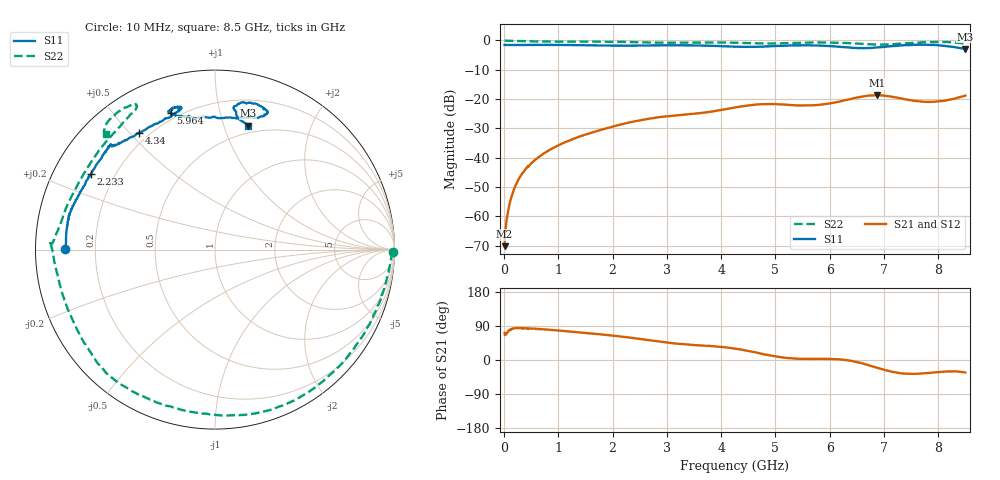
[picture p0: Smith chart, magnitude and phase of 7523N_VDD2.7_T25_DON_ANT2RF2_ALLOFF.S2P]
!Agilent Technologies,E5071C,MY46417908,A.11.23
!Date: Wed Dec 09 17:50:29 2020
!Data & Calibration Information:
!Freq	S11:SOLT2(ON)	S21:SOLT2(ON)	S12:SOLT2(ON)	S22:SOLT2(ON)
!PortZ  Port1:50+j0  Port2:50+j0
!Above PortZ is port z conversion or system Z0 setting when saving the data.
!When reading, reference impedance value at option line is always used.
# Hz S dB R 50
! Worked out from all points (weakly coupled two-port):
!   1601 points, 10 MHz to 8.5 GHz, reference 50 ohm
!   highest |S21| = -18.75 dB at 6.871 GHz (marker M1); lowest = -70.1 dB at 10 MHz (marker M2)
!   lowest |S11| = -2.9 dB at 8.5 GHz (marker M3), VSWR 6.02, Z = 21.4 + j60.4 ohm
!   |S11| at or under -10 dB: nowhere
!   |S22| runs from -1.5 to 0.0 dB; largest |S21 - S12| = 0.0013
!   S11 on the Smith chart (normalised r, x): 10 MHz: 0.09, +0.00; 2.233 GHz: 0.11, +0.28; 4.34 GHz: 0.16, +0.53; 5.964 GHz: 0.17, +0.72; 8.5 GHz: 0.43, +1.21
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1e7  -1.58 179.7  -70.15 71.3  -69.70 76.5  -0.05 -0.9
7.3675e7  -1.60 178.6  -58.28 74.8  -58.34 76.1  -0.15 -3.0
1.3735e8  -1.60 177.4  -53.30 81.1  -53.23 81.9  -0.19 -5.1
3.602125e8  -1.58 173.6  -44.87 83.4  -44.86 83.8  -0.30 -12.8
8.112438e8  -1.57 167.5  -37.62 80.2  -37.62 80.2  -0.42 -29.9
1.426769e9  -1.66 162.1  -32.56 72.3  -32.57 72.3  -0.45 -54.7
2.233319e9  -1.84 148.7  -28.32 60.5  -28.31 60.6  -0.56 -78.1
2.843538e9  -1.73 137.3  -26.23 48.8  -26.22 48.9  -0.78 -98.8
3.459062e9  -1.73 135.0  -25.08 40.0  -25.08 40.0  -0.78 -120.7
4.255e9  -2.20 125.4  -22.88 29.9  -22.87 29.8  -0.82 -136.2
4.3399e9  -2.21 123.2  -22.65 28.1  -22.62 28.1  -0.88 -138.2
5.003181e9  -1.95 104.5  -21.75 9.5  -21.72 9.6  -1.06 -165.2
5.3587e9  -1.76 103.9  -22.14 3.6  -22.13 3.8  -0.91 -178.2
5.671769e9  -1.75 107.5  -22.16 2.8  -22.14 3.3  -0.78 177.7
5.963612e9  -1.93 107.8  -21.62 2.9  -21.62 3.1  -0.76 177.8
6.4624e9  -2.60 95.6  -19.64 -4.3  -19.66 -4.1  -1.06 173.6
6.870981e9  -2.44 76.7  -18.75 -20.3  -18.79 -20.2  -1.47 152.0
7.088538e9  -2.08 70.5  -19.02 -29.0  -19.08 -29.1  -1.38 136.2
7.412219e9  -1.62 70.1  -20.20 -36.0  -20.17 -36.0  -0.99 120.7
7.666919e9  -1.47 74.0  -20.84 -35.8  -20.83 -35.8  -0.72 118.6
8.149788e9  -1.98 82.6  -20.48 -30.3  -20.48 -30.1  -0.61 128.5
8.5e9  -2.92 75.2  -18.85 -32.9  -18.84 -32.4  -1.08 133.4
